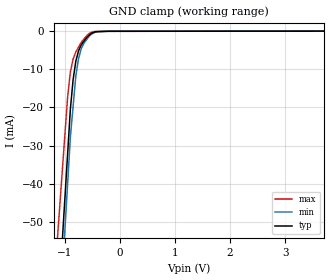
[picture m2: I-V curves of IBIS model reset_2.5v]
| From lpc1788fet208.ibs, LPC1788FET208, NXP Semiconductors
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[Model] reset_2.5v
Model_type Input
Vinl = 750.000mV
Vinh = 1.75000V
C_comp 1.640pF 1.560pF 1.720pF
| variable typ   min   max
[Voltage Range] 2.50000V 2.40000V 2.60000V
[POWER Clamp Reference] 2.50000V 2.40000V 2.60000V
[GND Clamp Reference] 0.00000V 0.00000V 0.00000V
[Temperature Range]   25   85   -40
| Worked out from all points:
|   GND clamp passes 1 mA (typ) near -0.56 V on its own axis
[GND Clamp]
-2.5V     -397.2mA   -420.9mA   -327.8mA
-950mV    -32.26mA   -40.07mA   -17.34mA
-900mV    -20.49mA   -27.79mA   -10.72mA
-850mV    -12.7mA    -19.72mA   -7.321mA
-800mV    -7.838mA   -11.65mA   -5.435mA
-750mV    -5.1mA     -7.135mA   -4.152mA
-700mV    -3.517mA   -4.495mA   -2.868mA
-650mV    -2.567mA   -3.047mA   -2.001mA
-550mV    -928.4uA   -1.201mA   -534.7uA
-400mV    -142.6uA   -110.2uA   -62.48uA
-200mV    -36.16uA   -30.1uA    -38.28uA
5V        17.06uA    15.81uA    16.52uA
[POWER Clamp]
-2.5V     0A         0A         0A
5V        0A         0A         0A
